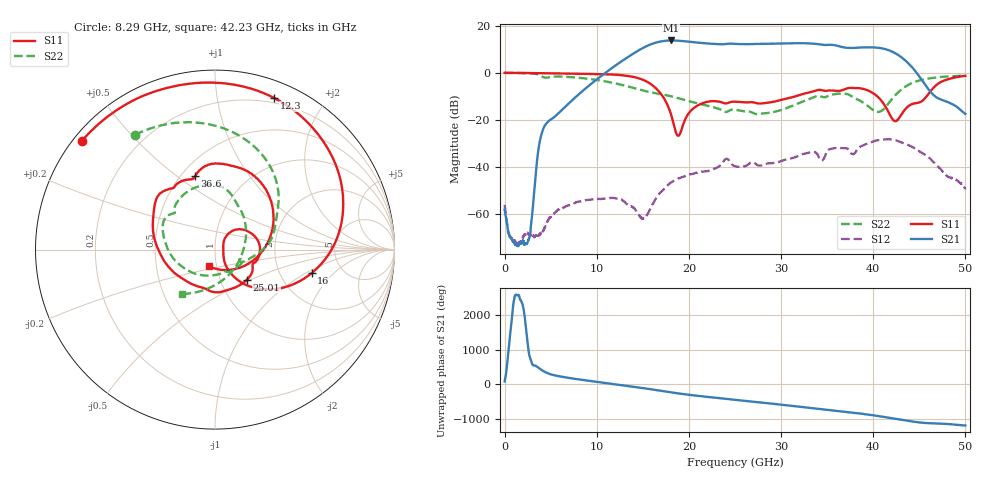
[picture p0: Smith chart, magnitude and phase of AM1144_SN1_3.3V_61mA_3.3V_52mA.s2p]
!Agilent Technologies,E8364B,MY43040894,A.07.50.67
!Agilent E8364B: A.07.50.67
!Date: Monday, November 15, 2021 11:02:37
!Correction: S11(Full 2 Port(1,2))
!S21(Full 2 Port(1,2))
!S12(Full 2 Port(1,2))
!S22(Full 2 Port(1,2))
!S2P File: Measurements: S11, S21, S12, S22:
# Hz S  dB  R 50
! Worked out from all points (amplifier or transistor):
!   6401 points, 10 MHz to 50 GHz, reference 50 ohm
!   highest |S21| = 13.8 dB at 18.06 GHz (marker M1)
!   |S21| within 3 dB of that: 15.11 GHz to 36.87 GHz (21.76 GHz wide, 83.7 % of centre)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
!   unconditionally stable (mu >= 1): 1.064 GHz to end of sweep
!   at 8.336 GHz: K = 22.35, MAG = 6.7 dB, |S12| = -54.5 dB
!   at 25 GHz: K = 10.64, MAG = 12.7 dB, |S12| = -39.6 dB
!   at 50 GHz: K = 62.99, MAG = -5.1 dB, |S12| = -49.2 dB
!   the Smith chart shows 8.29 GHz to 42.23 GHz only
!   S11 on the Smith chart (normalised r, x): 8.29 GHz: 0.02, +0.36; 12.3 GHz: 0.15, +1.45; 16 GHz: 3.01, -1.14; 25.01 GHz: 1.34, -0.48; 36.6 GHz: 0.58, +0.59; 42.23 GHz: 0.92, -0.17
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1e7  0.01 -3.7  -58.10 79.5  -56.07 46.7  -0.02 -4.2
8.289594e9  -0.38 140.6  -8.29 132.5  -54.47 47.2  -2.17 124.9
8.34427e9  -0.38 139.6  -8.11 130.5  -54.45 45.6  -2.19 123.9
1.230442e10  -0.85 68.6  3.88 -7.8  -53.53 -31.3  -4.70 61.8
1.404625e10  -1.77 33.3  8.36 -70.6  -57.45 -90.2  -6.48 41.8
1.599899e10  -5.13 -13.7  12.31 -148.6  -56.14 116.3  -8.36 26.5
1.667854e10  -7.57 -31.1  13.11 -176.8  -51.81 79.6  -8.85 21.6
1.806108e10  -17.58 -56.7  13.77 127.1  -46.56 31.4  -9.92 10.6
1.942799e10  -21.37 48.6  13.47 77.0  -44.08 -8.4  -11.38 0.6
2.134948e10  -13.11 24.4  12.70 16.1  -41.98 -54.2  -13.33 -10.3
2.5005e10  -12.24 -43.0  12.30 -86.8  -39.58 -153.8  -15.67 -30.6
2.501281e10  -12.24 -43.2  12.30 -87.1  -39.58 -153.8  -15.68 -30.7
2.882455e10  -12.53 -131.7  12.37 168.0  -38.33 123.4  -16.89 -92.7
3.126937e10  -10.27 -175.7  12.57 98.0  -36.11 64.4  -13.97 -148.9
3.333927e10  -8.04 149.8  12.44 34.9  -33.62 3.0  -10.70 166.9
3.512016e10  -7.52 121.1  11.94 -17.8  -32.67 -21.3  -9.75 134.0
3.659643e10  -7.42 105.0  11.00 -65.5  -31.93 -71.3  -8.79 101.1
3.979892e10  -8.18 33.9  10.85 -164.2  -29.40 -132.7  -15.25 13.4
4.167354e10  -16.81 -51.0  9.65 119.2  -28.17 165.5  -12.91 -102.6
4.222812e10  -20.25 -109.8  8.69 94.8  -28.41 145.1  -10.22 -126.7
4.487602e10  -12.68 24.4  -0.85 -13.6  -32.94 55.8  -3.37 161.8
5e10  -1.26 154.5  -17.42 -104.5  -49.24 -54.1  -1.15 101.2
